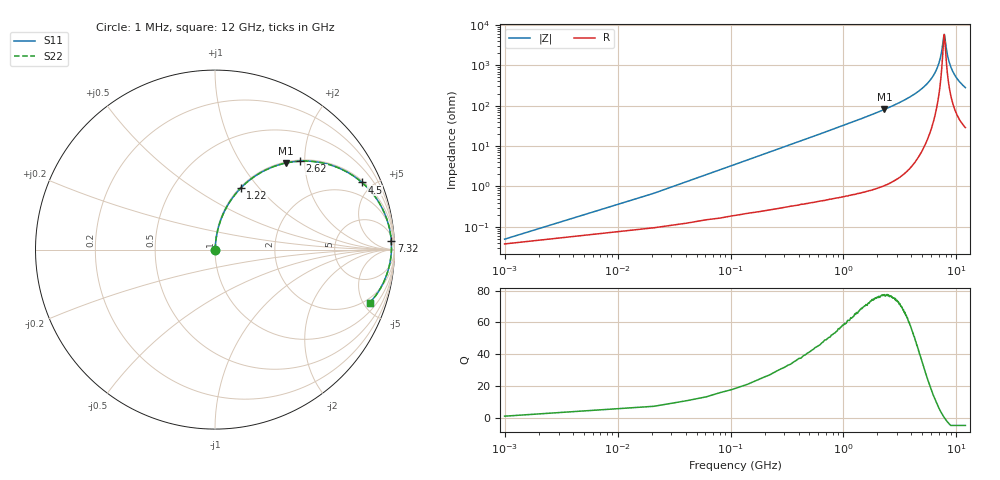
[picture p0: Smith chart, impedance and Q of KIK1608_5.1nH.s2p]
!version-2
!date-01.2022
!Series
# MHz S RI R 50
!Freq ReS11 ImS11 ReS21 ImS21 ReS12 ImS12 ReS22 ImS22
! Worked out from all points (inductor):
!   601 points, 1 MHz to 12 GHz, reference 50 ohm
!   read as one part in series: L = 5.1 nH near 61 MHz
!   highest Q = 77.1 at 2.3 GHz (marker M1), where L = 5.59 nH
!   self-resonance near 7.796 GHz
!   S11 on the Smith chart (normalised r, x): 1 MHz: 1.00, +0.00; 1.22 GHz: 1.01, +0.80; 2.62 GHz: 1.02, +1.89; 4.5 GHz: 1.10, +4.33; 7.32 GHz: 12, +36; 12 GHz: 1.57, -5.58
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1  0.000355 0.00032  0.9996 -0.00032  0.9996 -0.00032  0.000355 0.00032
81  0.00233 0.0259  0.9977 -0.0259  0.9977 -0.0259  0.00233 0.0259
141  0.00416 0.0449  0.9958 -0.0449  0.9958 -0.0449  0.00416 0.0449
241  0.00863 0.0764  0.9914 -0.0764  0.9914 -0.0764  0.00863 0.0764
401  0.0196 0.1259  0.9804 -0.1259  0.9804 -0.1259  0.0196 0.1259
601  0.04 0.1852  0.96 -0.1852  0.96 -0.1852  0.04 0.1852
1220  0.1425 0.3418  0.8575 -0.3418  0.8575 -0.3418  0.1425 0.3418
2020  0.3274 0.4627  0.6726 -0.4627  0.6726 -0.4627  0.3274 0.4627
2300  0.3962 0.4827  0.6038 -0.4827  0.6038 -0.4827  0.3962 0.4827
2620  0.4732 0.4928  0.5268 -0.4928  0.5268 -0.4928  0.4732 0.4928
4020  0.7512 0.4234  0.2488 -0.4234  0.2488 -0.4234  0.7512 0.4234
4500  0.8186 0.3744  0.1814 -0.3744  0.1814 -0.3744  0.8186 0.3744
6020  0.9474 0.1957  0.0526 -0.1957  0.0526 -0.1957  0.9474 0.1957
6800  0.9746 0.1054  0.0254 -0.1054  0.0254 -0.1054  0.9746 0.1054
7320  0.9822 0.0488  0.0178 -0.0488  0.0178 -0.0488  0.9822 0.0488
7760  0.9832 0.00362  0.0168 -0.00362  0.0168 -0.00362  0.9832 0.00362
7860  0.9829 -0.00627  0.0171 0.00627  0.0171 0.00627  0.9829 -0.00627
8020  0.9819 -0.0218  0.0181 0.0218  0.0181 0.0218  0.9819 -0.0218
8320  0.9788 -0.0499  0.0212 0.0499  0.0212 0.0499  0.9788 -0.0499
8720  0.9724 -0.0854  0.0276 0.0854  0.0276 0.0854  0.9724 -0.0854
10020  0.938 -0.1851  0.062 0.1851  0.062 0.1851  0.938 -0.1851
12000  0.8637 -0.2956  0.1363 0.2956  0.1363 0.2956  0.8637 -0.2956
